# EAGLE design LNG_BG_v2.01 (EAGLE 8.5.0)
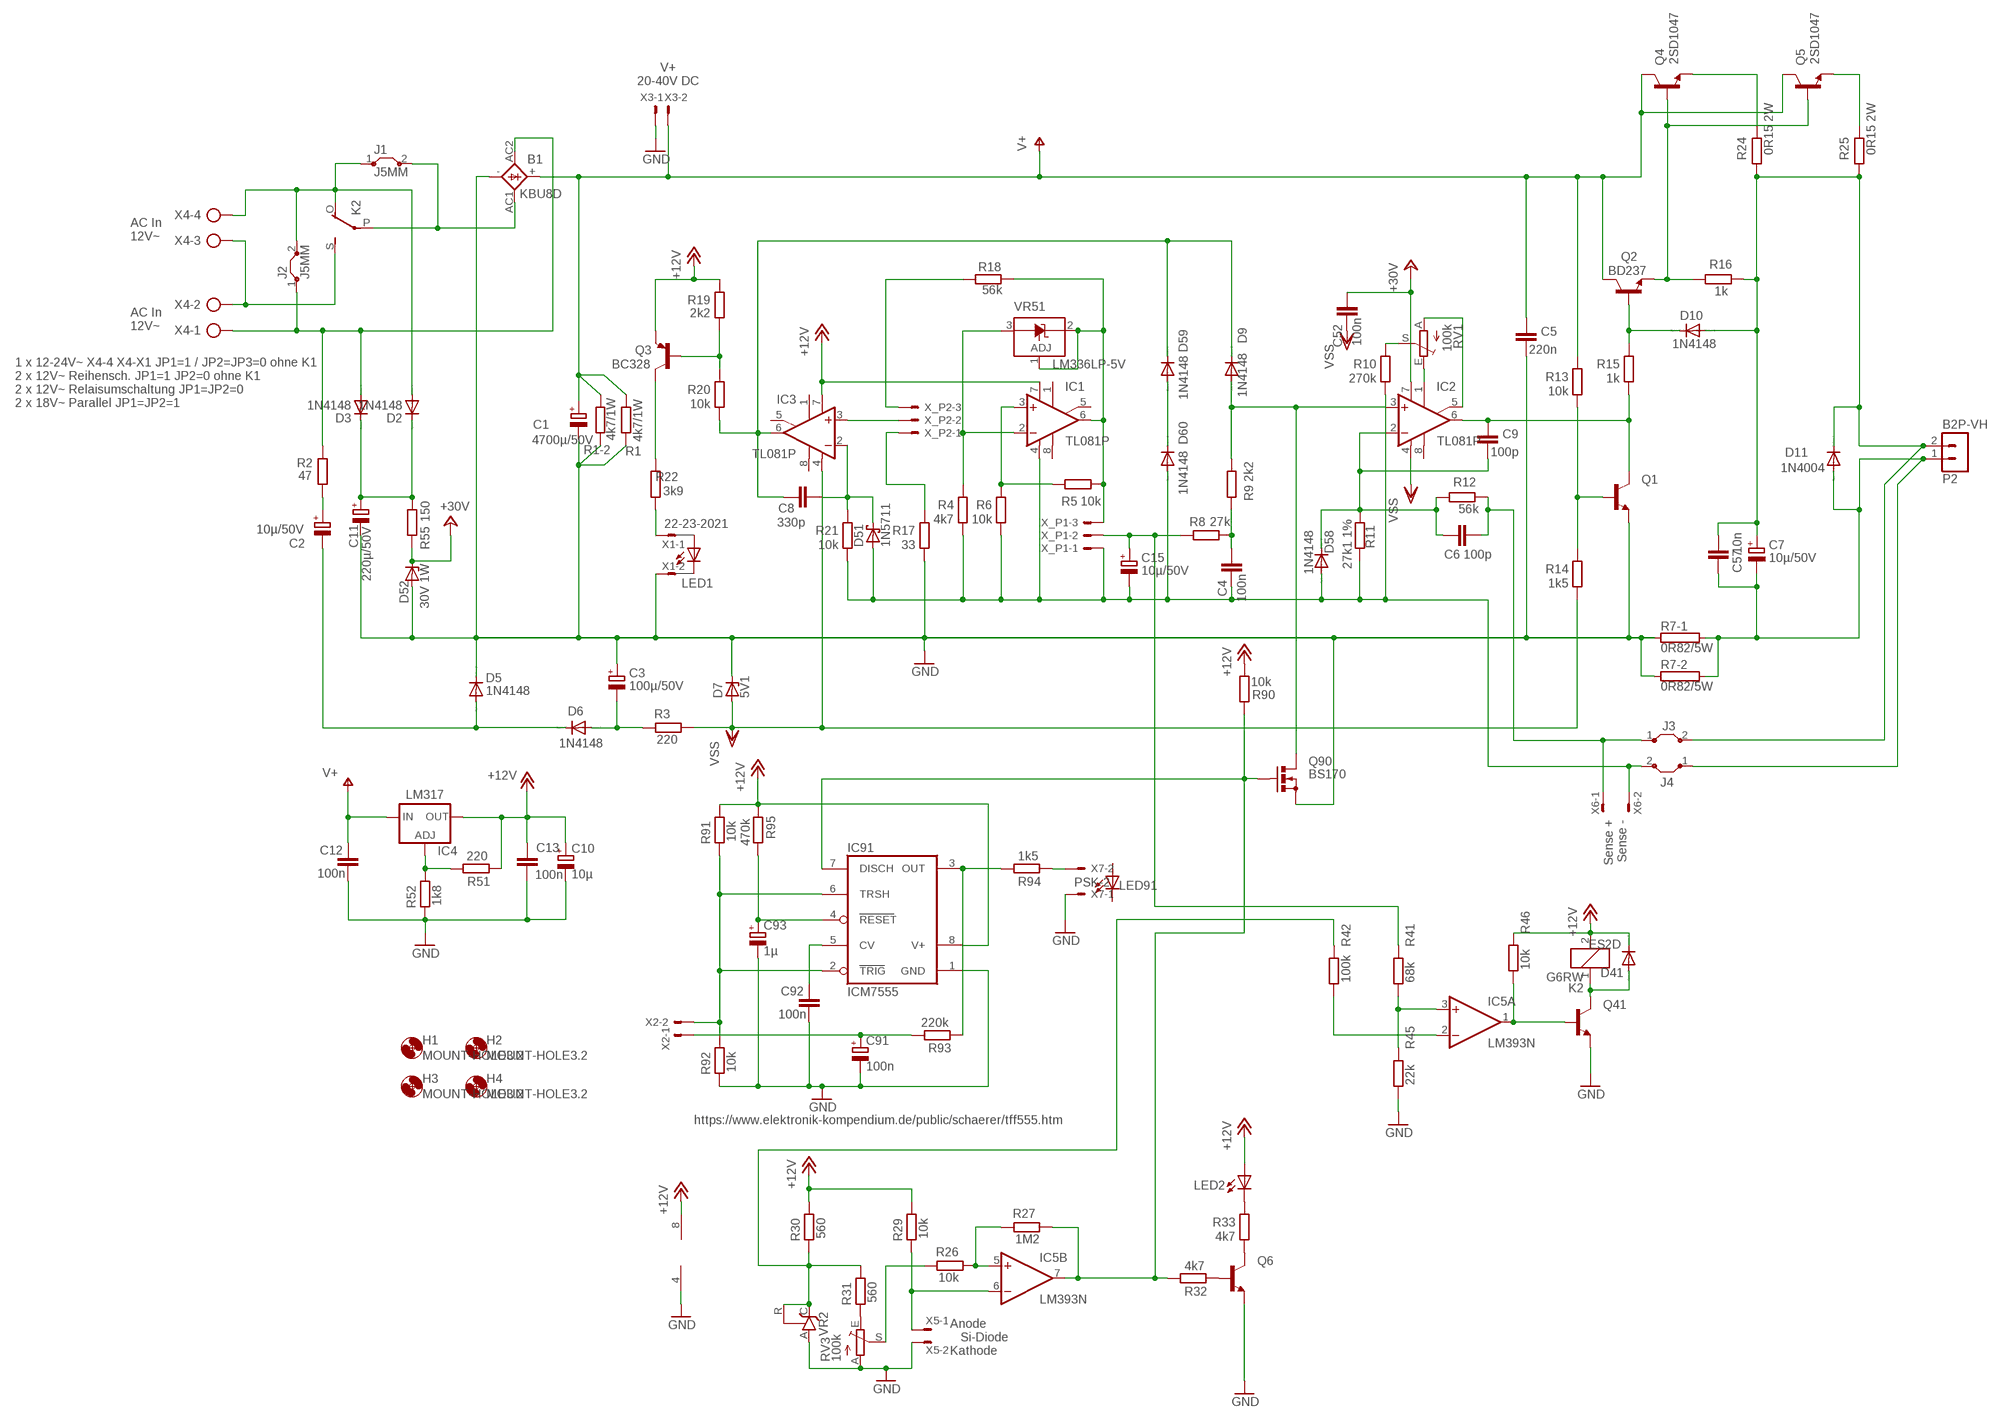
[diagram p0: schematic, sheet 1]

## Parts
B1  KBU8D  GBU4  [GBU4S]
C1  4700µ/50V  CPOL-EUE10-25  [EB25D]
C2  10µ/50V  CPOL-EUE2.5-6  [E2,5-6]
C3  100µ/50V  CPOL-EUE2.5-6  [E2,5-6]
C4  100n  C-EU050-024X044  [C050-024X044]
C5  220n  C-EUC1206  [C1206]
C6  100p  C-EU050-024X044  [C050-024X044]
C7  10µ/50V  CPOL-EUE2.5-6  [E2,5-6]
C8  330p  C-EU050-024X044  [C050-024X044]
C9  100p  C-EU050-024X044  [C050-024X044]
C10  10µ  CPOL-EUE1.8-4  [E1,8-4]
C11  220µ/50V  CPOL-EUE5-10.5  [E5-10,5]
C12  100n  C-EUC0805K  [C0805K]
C13  100n  C-EUC0805K  [C0805K]
C15  10µ/50V  CPOL-EUE2.5-6  [E2,5-6]
C52  100n  C-EUC1206K  [C1206K]
C57  10n  C-EU050-024X044  [C050-024X044]
C91  100n  CPOL-EUE1.8-4  [E1,8-4]
C92  100n  C-EU050-024X044  [C050-024X044]
C93  1µ  CPOL-EUE1.8-4  [E1,8-4]
D2  1N4148  1N4004  [DO41-10]
D3  1N4148  1N4004  [DO41-10]
D5  1N4148  1N4148DO35-10  [DO35-10]
D6  1N4148  1N4148DO35-10  [DO35-10]
D7  5V1  BZV10  [DO34Z7]
D9  1N4148  1N4148DO35-10  [DO35-10]
D10  1N4148  1N4148DO35-10  [DO35-10]
D11  1N4004  [DO41-10]
D41  ES2D  [SMB]
D51  1N5711  SCHOTTKY-DIODEDO35-7  [DO35-7]
D52  30V 1W  ZPY  [DO41Z10]
D58  1N4148  1N4148DO35-10  [DO35-10]
D59  1N4148  1N4148DO35-10  [DO35-10]
D60  1N4148  1N4148DO35-10  [DO35-10]
H1  MOUNT-HOLE3.2  [3,2]
H2  MOUNT-HOLE3.2  [3,2]
H3  MOUNT-HOLE3.2  [3,2]
H4  MOUNT-HOLE3.2  [3,2]
IC1  TL081P  [DIL08]
IC2  TL081P  [DIL08]
IC3  TL081P  [DIL08]
IC4  LM317  LM317TS  [317TS]
IC5  LM393N  [DIL08]
IC91  ICM7555  [DIL08]
J1  J5MM  [05]
J2  J5MM  [05]
J3  J5MM  [05]
J4  J5MM  [05]
K2  G6RW  [G6RW]
LED1  LED3MM  [LED3MM]
LED2  LED3MM  [LED3MM]
LED91  LED3MM  [LED3MM]
P2  B2P-VH  [B2P-VH]
Q1  BC337-NPN-TO92-CBE  [TO92-CBE]
Q2  BD237  -NPN-TO126V  [TO126V]
Q3  BC328  [TO92-EBC]
Q4  2SD1047  2SC3855  [SC-65]
Q5  2SD1047  2SC3855  [SC-65]
Q6  BC337-NPN-TO92-CBE  [TO92-CBE]
Q41  BC337-NPN-TO92-CBE  [TO92-CBE]
Q90  BS170  [SOT54E]
R1  4k7/1W  R-EU_R2512  [R2512]
R1-2  4k7/1W  R-EU_R2512  [R2512]
R2  47  R-EU_0207/10  [0207/10]
R3  220  R-EU_0207/10  [0207/10]
R4  4k7  R-EU_0207/10  [0207/10]
R5  10k  R-EU_0207/10  [0207/10]
R6  10k  R-EU_0207/10  [0207/10]
R7-1  0R82/5W  RKH208-8  [KH208-8]
R7-2  0R82/5W  RKH208-8  [KH208-8]
R8  27k  R-EU_0207/10  [0207/10]
R9  2k2  R-EU_0207/10  [0207/10]
R10  270k  R-EU_0207/10  [0207/10]
R11  27k1 1%  R-EU_0207/10  [0207/10]
R12  56k  R-EU_0207/10  [0207/10]
R13  10k  R-EU_0207/10  [0207/10]
R14  1k5  R-EU_0207/10  [0207/10]
R15  1k  R-EU_0207/10  [0207/10]
R16  1k  R-EU_0207/10  [0207/10]
R17  33  R-EU_0207/10  [0207/10]
R18  56k  R-EU_0207/10  [0207/10]
R19  2k2  R-EU_0207/10  [0207/10]
R20  10k  R-EU_0207/10  [0207/10]
R21  10k  R-EU_0207/10  [0207/10]
R22  3k9  R-EU_0207/10  [0207/10]
R24  0R15 2W  R-EU_0613/15  [P0613/15]
R25  0R15 2W  R-EU_0613/15  [P0613/15]
R26  10k  R-EU_0207/10  [0207/10]
R27  1M2  R-EU_0207/10  [0207/10]
R29  10k  R-EU_0207/10  [0207/10]
R30  560  R-EU_0207/10  [0207/10]
R31  560  R-EU_0207/10  [0207/10]
R32  4k7  R-EU_0207/10  [0207/10]
R33  4k7  R-EU_0207/10  [0207/10]
R41  68k  R-EU_0207/10  [0207/10]
R42  100k  R-EU_0207/10  [0207/10]
R45  22k  R-EU_0207/10  [0207/10]
R46  10k  R-EU_0207/10  [0207/10]
R51  220  R-EU_0207/10  [0207/10]
R52  1k8  R-EU_0207/10  [0207/10]
R55  150  R-EU_0207/10  [0207/10]
R90  10k  R-EU_0207/10  [0207/10]
R91  10k  R-EU_0207/10  [0207/10]
R92  10k  R-EU_0207/10  [0207/10]
R93  220k  R-EU_0207/10  [0207/10]
R94  1k5  R-EU_0207/10  [0207/10]
R95  470k  R-EU_0207/10  [0207/10]
RV1  100k  TRIM_EU-B64Y  [B64Y]
RV3  100k  TRIM_EU-B64Y  [B64Y]
VR2  TL431CLP  [TO92-CLP]
VR51  LM336LP-5V  LM336LP  [TO92]
X1  22-23-2021  [22-23-2021]
X2  PSK-2  22-23-2021  [22-23-2021]
X3  PSK-2  22-23-2021  [22-23-2021]
X4  AK500/4  [AK500/4]
X5  PSK-2  22-23-2021  [22-23-2021]
X6  22-23-2021  [22-23-2021]
X7  PSK-2  22-23-2021  [22-23-2021]
X_P1  22-23-2031  [22-23-2031]
X_P2  22-23-2031  [22-23-2031]

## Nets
+12V: C10.+ C13.1 D41.C IC1.7(V+) IC3.7(V+) IC4.2(OUT) IC5.8(P:V+) IC91.8(V+) K2.2 LED2.A Q3.E R19.2 R29.2 R30.2 R46.2 R51.1 R90.1 R91.2 R95.1
+24V: C52.1 D52.C IC2.7(V+) R55.1 ; supply symbol labelled +30V
+SENSE: C7.+ C57.2 D10.A D11.C J3.2 P2.2 R16.1 R24.2 R25.2
-SENSE: C4.2 C15.- D51.A D58.A D60.A IC1.4(V-) J4.2 R4.1 R6.1 R10.1 R11.1 R21.1 X6.2 X_P1.1
AC2-1: K2.S(2:S) X4.2 X4.3
AC2-2: B1.AC2(AC1) D3.A J2.1 R2.1 X4.1
GND: B1.- C1.- C3.+ C5.2 C10.- C11.- C12.2 C13.2 C91.- C92.2 C93.- D5.C D7.C D52.A IC5.4(P:V-) IC91.1(GND) Q1.E Q6.E Q41.E Q90.S R1-2.1 R1.1 R7-1.1 R7-2.1 R17.1 R45.1 R52.1 R92.1 RV3.A VR2.A X1.2 X3.1 X5.2 X7.1
N$1: IC91.3(OUT) R93.1 R94.2
N$2: R94.1 X7.2
N$3: C2.+ R2.2
N$4: B1.AC1(AC2) J1.2 K2.P(2:P)
N$5: C2.- D5.A D6.C
N$6: Q3.B R19.1 R20.2
N$7: C3.- D6.A R3.1
N$8: D59.A D60.C
N$9: C8.2 D9.C D59.C IC3.6(OUT) R20.1
N$10: C8.1 D51.C IC3.2(-IN) R21.2
N$11: R22.1 X1.1
N$12: Q3.C R22.2
N$13: C11.+ D2.C D3.C R55.2
N$14: IC3.3(+IN) X_P2.2
N$15: R17.2 X_P2.1
N$16: R18.2 X_P2.3
N$17: IC1.3(+IN) R5.2 R6.2
N$18: C15.+ R8.2 R41.2 X_P1.2
N$19: IC1.2(-IN) R4.2 VR51.3(A)
N$21: C4.1 R8.1 R9.2
N$22: D9.A IC2.3(+IN) Q90.D R9.1
N$23: C93.+ IC91.4(RESET) R95.2
N$24: R10.2 RV1.S
N$25: IC2.1(ON1) RV1.E
N$26: IC2.5(ON2) RV1.A
N$27: C9.1 IC2.6(OUT) Q1.C R15.1
N$28: Q1.B R13.1 R14.2
N$29: D10.C Q2.3(B) R15.2
N$30: IC5.3(A:+IN) R41.1 R45.2
N$31: IC5.5(B:+IN) R26.2 R27.1
N$32: IC91.2(TRIG) IC91.6(TRSH) R91.1 R92.2 X2.2
N$33: IC5.2(A:-IN) R42.1
N$35: C6.1 C9.2 D58.C IC2.2(-IN) R11.2 R12.2
N$36: C92.1 IC91.5(CV)
N$37: IC5.6(B:-IN) R29.1 X5.1
N$39: IC5.1(A:OUT) Q41.B R46.1
N$40: R30.1 R31.2 R42.2 VR2.C VR2.R
N$41: D41.A K2.1 Q41.C
N$42: Q4.3(E) R24.1
N$43: R31.1 RV3.E
N$44: IC4.1(ADJ) R51.2 R52.2
N$45: R26.1 RV3.S
N$46: D2.A J1.1 J2.2 K2.O(2:O) X4.4
N$48: C6.2 J3.1 R12.1 X6.1
N$50: Q2.1(E) Q4.1(B) Q5.1(B) R16.2
N$51: Q5.3(E) R25.1
N$53: C91.+ R93.2 X2.1
N$54: Q6.B R32.1
N$55: C7.- C57.1 D11.A J4.1 P2.1 R7-1.2 R7-2.2
N$56: Q6.C R33.1
N$57: LED2.K(C) R33.2
N$58: IC5.7(B:OUT) IC91.7(DISCH) Q90.G R27.2 R32.2 R90.2
V+: B1.+ C1.+ C5.1 C12.1 IC4.3(IN) Q2.2(C) Q4.2(C) Q5.2(C) R1-2.2 R1.2 R13.2 X3.2
VREF: IC1.6(OUT) R5.1 R18.1 VR51.1(ADJ) VR51.2(C) X_P1.3
VSS: C52.2 D7.A IC2.4(V-) IC3.4(V-) R3.2 R14.1
Unconnected: IC1.1(ON1) IC1.5(ON2) IC1.8(OPT) IC2.8(OPT) IC3.1(ON1) IC3.5(ON2) IC3.8(OPT) LED1.A LED1.K(C) LED91.A LED91.K(C)

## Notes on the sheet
- V+
  20-40V DC
- AC In
  12V~
- AC In
  12V~
- 1 x 12-24V~ X4-4 X4-X1 JP1=1 / JP2=JP3=0 ohne K1
  2 x 12V~ Reihensch. JP1=1 JP2=0 ohne K1
  2 x 12V~ Relaisumschaltung JP1=JP2=0
  2 x 18V~ Parallel JP1=JP2=1
- Sense +
  Sense -
- https://www.elektronik-kompendium.de/public/schaerer/tff555.htm
- Anode
     Si-Diode
  Kathode

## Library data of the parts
B1 = rectifier:GBU4: GENERAL INSTRUMENT RECTIFIER
C1-C3 C7 C10 C11 C15 C91 C93 = rcl:CPOL-EU: POLARIZED CAPACITOR, European symbol; SPICEPREFIX: C
C4-C6 C8 C9 C12 C13 C52 C57 C92 = rcl:C-EU: CAPACITOR, European symbol; SPICEPREFIX: C
D2 D3 D11 = diode:1N4004: DIODE
D5 D6 D9 D10 D58-D60 = diode:1N4148: DIODE
D7 = diode:BZV10: Z DIODE
D41 = diode:ES2D: DIODE
D51 = diode:SCHOTTKY-DIODE: Schottky Diode
D52 = diode:ZPY: Z DIODE
H1-H4 = holes:MOUNT-HOLE: MOUNTING HOLE with drill center marker
IC1-IC3 = linear:TL081: OP AMP
IC4 = v-reg:LM317TS: VOLTAGE REGULATOR
IC5 = linear:LM393: COMPARATOR
IC91 = maxim:ICM7555: TIMER; MF: MAXIM; MPN: ICM7555IPA+; OC_FARNELL: 9663762; OC_NEWARK: 68K4387
J1-J4 = jumper:J: Bridge
K2 = relay:G6RW: RELAY 1 x switch, Omron; OC_FARNELL: unknown; OC_NEWARK: unknown
LED1 LED2 LED91 = led:LED: LED
P2 = con-jst-vh:B2P-VH: HEADER
Q1 Q2 Q6 Q41 = transistor:*-NPN-: NPN Transistror BF959 corrected 2008.03.06
Q3 = transistor-pnp:BC328*: PNP Transistror
Q4 Q5 = transistor-JP:2SC3855: NPN Power Transistor 140V, 10A, 100W
Q90 = transistor-small-signal:BS170: N-CHANNEL MOS FET
R1 R1-2 R2-R6 R8-R22 R24-R27 R29-R33 R41 R42 R45 R46 R51 R52 R55 R90-R95 = rcl:R-EU_: RESISTOR, European symbol; SPICEPREFIX: R
R7-1 R7-2 = resistor-power:R: Power Resitor; OC_FARNELL: unknown; OC_NEWARK: unknown
RV1 RV3 = pot:TRIM_EU-: POTENTIOMETER
VR2 = v-reg:TL431CLP: VOLTAGE REGULATOR
VR51 = linear:LM336: 2.5-V INTEGRATED REFERENCE CIRCUITS LM236 Source: http://focus.ti.com/lit/ds/symlink/lm336-2.5.pdf
X1-X3 X5-X7 = con-molex:22-23-2021: .100" (2.54mm) Center Header - 2 Pin; MF: MOLEX; MPN: 22-23-2021; OC_FARNELL: 1462926; OC_NEWARK: 25C3832
X4 = con-ptr500:AK500/4: CONNECTOR; OC_FARNELL: unknown; OC_NEWARK: unknown
X_P1 X_P2 = con-molex:22-23-2031: .100" (2.54mm) Center Header - 3 Pin; MF: MOLEX; MPN: 22-23-2031; OC_FARNELL: 1462950; OC_NEWARK: 30C0862

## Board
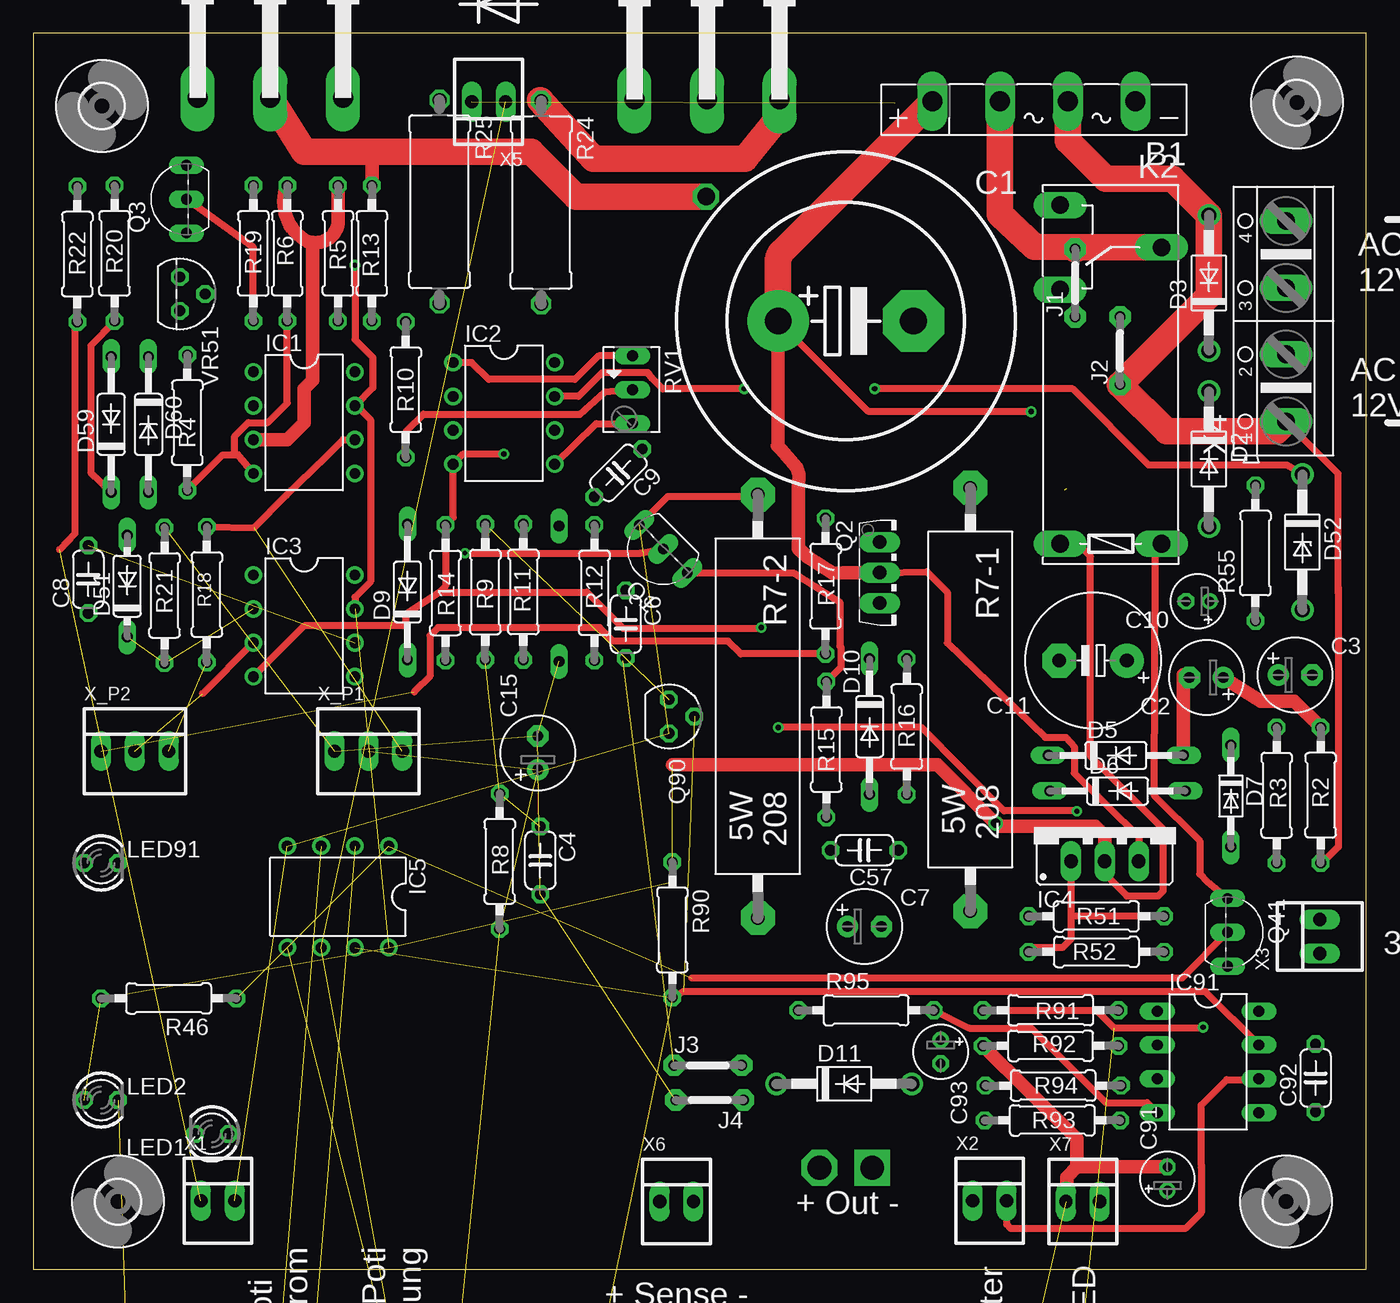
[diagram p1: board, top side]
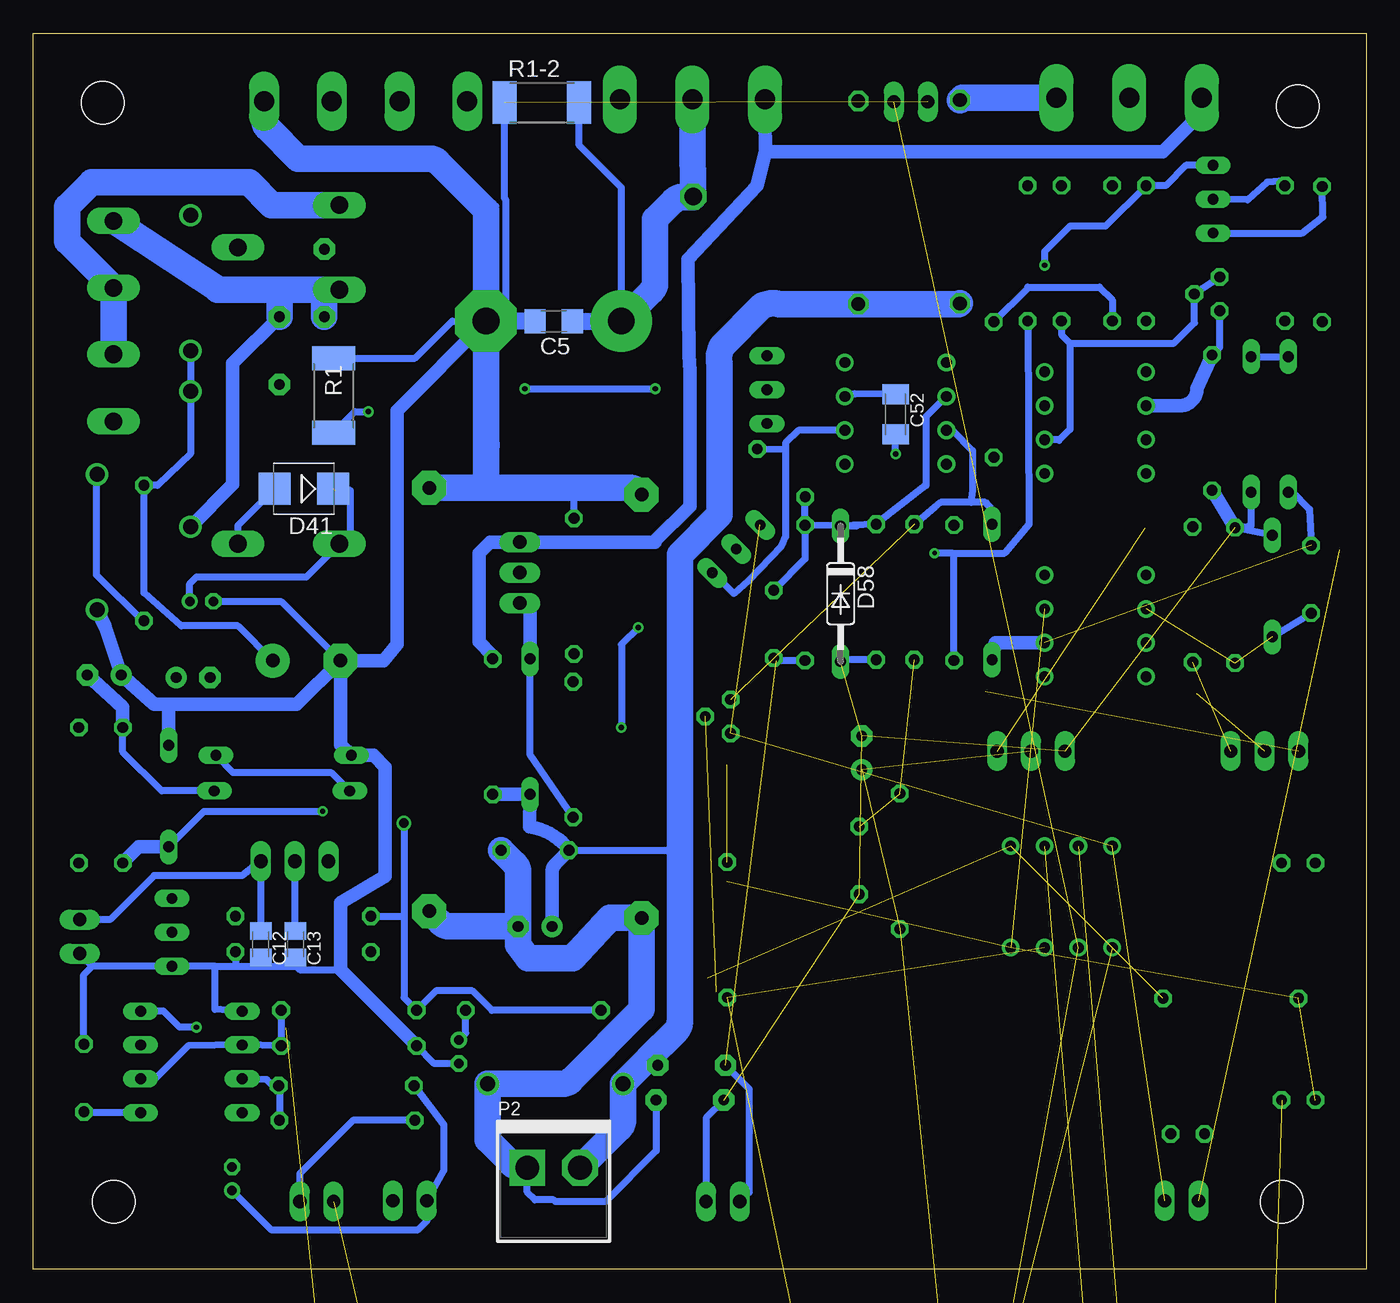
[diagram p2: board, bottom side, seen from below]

Size 100 x 92.7 mm. Coordinates in mm from the lower left corner, seen from the top.
Outline: 0,0 100,0 100,92.7 0,92.7 0,0
Copper layers (1*16): Top 0.035mm / dielectric 1.5mm / Bottom 0.035mm
Design rules "default *": minimum track width 6mil, minimum drill 0.35mm, track to track 10mil, track to pad 10mil, pad to pad 10mil, via to via 15mil, smd to smd 6mil, copper to edge 40mil, drill to drill 6mil, minimum pad ring 10mil, minimum via ring 8mil, stop-mask expansion 4mil, vias tented up to drill 0mil, thermal gap 10mil

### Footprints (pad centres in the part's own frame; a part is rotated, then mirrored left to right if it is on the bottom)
GBU4S = drill 1.499 long: + 7.62,0; - -7.62,0; AC1 2.54,0; AC2 -2.54,0
EB25D = drill 2.007 pad 4.597: + -5.08,0 | drill 2.007 pad 4.597 octagon: - 5.08,0
E2,5-6 = drill 0.813 pad 1.6: + -1.27,0 | drill 0.813 pad 1.6 octagon: - 1.27,0
C050-024X044 = drill 0.813 octagon: 1 -2.54,0; 2 2.54,0
C1206 = smd 1.6 x 1.8: 1 -1.4,0; 2 1.4,0
E1,8-4 = drill 0.711 pad 1.168: + -0.889,0 | drill 0.711 pad 1.168 octagon: - 0.889,0
E5-10,5 = drill 1.016 pad 2.54: + -2.54,0 | drill 1.016 pad 2.54 octagon: - 2.54,0
C0805K = smd 1.3 x 1.6: 1 -1,0; 2 1,0
C1206K = smd 1.5 x 2: 1 -1.5,0; 2 1.5,0
DO41-10 = drill 1.118: A 5.08,0; C -5.08,0
DO35-10 = drill 0.813 long: A 5.08,0; C -5.08,0
DO34Z7 = drill 0.813 long: A 3.81,0; C -3.81,0
SMB = smd 2.4 x 2.4: A 2.2,0; C -2.2,0
DO35-7 = drill 0.813 long: A 3.81,0; C -3.81,0
DO41Z10 = drill 1.118: A 5.08,0; C -5.08,0
3,2 = hole 3.2: 0,0
DIL08 = drill 0.813 pad 1.27: 1 -3.81,-3.81; 2 -1.27,-3.81; 3 1.27,-3.81; 4 3.81,-3.81; 5 3.81,3.81; 6 1.27,3.81; 7 -1.27,3.81; 8 -3.81,3.81
317TS = drill 1.016 long: 1 -2.54,-2.54; 2 0,-2.54; 3 2.54,-2.54
DIL08' = drill 0.813 long: 1 -3.81,-3.81; 2 -1.27,-3.81; 3 1.27,-3.81; 4 3.81,-3.81; 5 3.81,3.81; 6 1.27,3.81; 7 -1.27,3.81; 8 -3.81,3.81
05 = drill 0.813 pad 1.6 octagon: 1 -2.54,0; 2 2.54,0
G6RW = drill 1.321 long: 1 -12.7,-3.81; 2 -12.7,3.81; O 6.35,3.81; P 9.525,-3.81; S 12.7,3.81
LED3MM = drill 0.813 octagon: A -1.27,0; K 1.27,0
B2P-VH = drill 1.778 square: 1 -1.98,0 | drill 1.778 octagon: 2 1.98,0
TO92-CBE = drill 0.813 long: B 0,0; C -2.54,0; E 2.54,0
TO126V = drill 1.016 long: 1 -2.286,-1.27; 2 0,-1.27; 3 2.286,-1.27
TO92-EBC = drill 0.813 long: B 0,-1.27; C -2.54,-1.27; E 2.54,-1.27
SC-65 = drill 1.5 pad 2.54 long: 1 -5.45,-18.81; 2 0,-18.81; 3 5.45,-18.81
SOT54E = drill 0.813 octagon: D -1.27,0; G 0,1.905; S 1.27,0
R2512 = smd 1.8 x 3.2: 1 -2.8,0; 2 2.8,0
0207/10 = drill 0.813 octagon: 1 -5.08,0; 2 5.08,0
KH208-8 = drill 1.016 pad 2.54 octagon: 1 -15.875,0; 2 15.875,0
P0613/15 = drill 1.016 octagon: 1 -7.62,0; 2 7.62,0
B64Y = drill 0.813 long: A 2.54,0; E -2.54,0; S 0,0
TO92-CLP = drill 0.813 octagon: A 0,1.905; C 1.27,0; R -1.27,0
TO92 = drill 0.813 octagon: 1 -1.27,0; 2 0,1.905; 3 1.27,0
22-23-2021 = drill 1 long: 1 -1.27,0; 2 1.27,0
AK500/4 = drill 1.321 long: 1 -7.518,0; 2 -2.489,0; 3 2.489,0; 4 7.518,0
22-23-2031 = drill 1 long: 1 -2.54,0; 2 0,0; 3 2.54,0

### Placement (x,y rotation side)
B1  75.07,87.61 180 top
C1  60.96,71.12 0 top
C2  88.01,44.39 180 top
C3  94.68,44.58 0 top
C4  38.04,30.67 270 top
C5  60.96,71.12 180 bottom
C6  44.45,48.39 270 top
C7  62.36,25.72 0 top
C8  4.13,51.75 90 top
C9  43.89,59.73 225 top
C10  87.38,50.1 180 top
C11  79.5,45.66 180 top
C12  82.93,24.38 270 bottom
C13  80.33,24.38 270 bottom
C15  37.85,38.73 90 top
C52  35.31,64.14 270 bottom
C57  62.36,31.43 180 top
C91  85.09,6.79 90 top
C92  96.2,14.35 90 top
C93  68.07,16.32 270 top
D2  88.2,60.77 270 top
D3  88.2,73.98 90 top
D5  81.22,38.54 0 top
D6  81.34,35.88 0 top
D7  89.85,35.5 270 top
D9  28.07,50.8 90 top
D10  62.74,40.7 270 top
D11  60.83,13.91 0 top
D41  79.69,58.55 180 bottom
D51  7.05,51.24 90 top
D52  95.21,54.54 270 top
D58  39.43,50.67 270 bottom
D59  5.84,63.37 90 top
D60  8.64,63.37 270 top
H1  5.14,87.25 0 top
H2  6.35,5.08 0 top
H3  93.98,5.08 0 top
H4  94.81,87.5 0 top
IC1  20.32,63.5 270 top
IC2  35.31,64.2 270 top
IC3  20.32,48.26 270 top
IC4  80.39,33.15 0 top
IC5  22.86,27.94 180 top
IC91  ICM7555  [DIL08']  88.14,15.56 270 top
J1  78.17,73.98 90 top
J2  81.53,68.9 90 top
J3  50.61,15.3 0 top
J4  50.74,12.7 180 top
K2  80.84,67.12 90 top
LED1  13.4,10.16 180 top
LED2  5.08,12.7 0 top
LED91  5.08,30.48 0 top
P2  60.96,7.62 0 bottom
Q1  47.26,54.03 135 top
Q2  64.77,52.26 270 top
Q3  10.22,80.26 90 top
Q4  50.55,106.55 0 top
Q5  17.78,106.68 0 top
Q6  not placed on the board
Q41  89.6,25.27 270 top
Q90  47.69,41.47 270 top
R1  77.47,65.53 270 bottom
R1-2  61.85,87.5 0 bottom
R2  96.58,35.56 90 top
R3  93.28,35.56 270 top
R4  11.56,63.5 90 top
R5  22.86,76.2 90 top
R6  19.05,76.2 90 top
R7-1  70.29,42.74 270 top
R7-2  54.36,42.23 270 top
R8  34.99,30.61 270 top
R9  33.91,50.8 270 top
R10  27.94,65.98 270 top
R11  36.77,50.8 90 top
R12  42.1,50.74 90 top
R13  25.4,76.2 90 top
R14  30.92,50.74 270 top
R15  59.5,38.99 270 top
R16  65.53,40.7 90 top
R17  59.44,51.24 270 top
R18  13.02,50.61 270 top
R19  16.51,76.2 90 top
R20  6.1,76.2 90 top
R21  9.84,50.55 270 top
R22  3.3,76.14 90 top
R24  38.1,80.01 270 top
R25  30.48,80.07 270 top
R26  not placed on the board
R27  not placed on the board
R29  not placed on the board
R30  not placed on the board
R31  not placed on the board
R32  not placed on the board
R33  not placed on the board
R41  not placed on the board
R42  not placed on the board
R45  not placed on the board
R46  10.16,20.32 180 top
R51  79.76,26.48 0 top
R52  79.76,23.81 180 top
R55  91.69,53.72 90 top
R90  47.94,25.46 270 top
R91  76.33,19.43 180 top
R92  76.33,16.76 0 top
R93  76.52,13.78 180 top
R94  76.45,11.18 0 top
R95  62.48,19.43 0 top
RV1  44.96,65.98 270 top
RV3  not placed on the board
VR2  not placed on the board
VR51  10.99,73.15 270 top
X1  13.84,5.14 0 top
X2  71.75,5.14 0 top
X3  96.52,24.96 90 top
X4  93.98,71.12 90 top
X5  34.16,87.57 180 top
X6  48.26,5.08 0 top
X7  78.74,5.08 0 top
X_P1  25.15,38.86 0 top
X_P2  7.62,38.86 0 top

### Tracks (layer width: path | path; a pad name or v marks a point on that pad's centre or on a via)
+12V  (via drill 0.4, 0.7)  (8 unrouted)
  Top 0.508: IC3.7 24.13,50.42 25.3,51.59 25.3,63.73 24.13,64.9 IC1.7 25.46,66.1 25.46,68.39 24.13,69.72 v24.13,75.31 | 47.94,29.08 R90.1 | R91.2 79.75,19.43 81.05,18.14 87.73,18.14 v87.76,18.16 | IC4.2 80.39,29.66 82.04,28 84.39,28 84.77,28.38 84.77,33.02 79.31,38.48 79.31,53.47 78.3,54.48 78.23,54.42 K2.2
  Top 1.016: IC4.2 80.39,32.51 79.69,33.21 72.57,33.21 72.32,33.46 v72.2,33.46 67.82,37.85 47.94,37.85
  Bottom 0.508: Q3.E 13.53,82.8 15.05,81.28 R19.2 19.56,78.23 22.23,78.23 24.13,76.33 v24.13,75.31 | 77.36,58.42 76.2,58.42 76.2,55.24 K2.2 79.5,51.94 87.76,51.94 88.27,51.43 C10.+ | 70.93,19.43 R91.2 | IC4.2 80.39,25.45 C13.1 | R91.2 72.2,20.38 72.2,26.42 | v72.2,33.46 72.2,26.42 | R95.1 65.6,19.43 67.06,20.89 69.79,20.89 R91.2 | v87.76,18.16 89.03,18.16 90.23,19.37 IC91.8 | R51.1 72.26,26.48 72.2,26.42
+24V  (via drill 0.4)
  Top 0.508: v53.34,66.04 47.21,66.04 46.46,66.78 46.1,67.25 42.67,67.25 40.89,65.47 IC2.7 | v63.12,66.04 77.98,66.04 83.69,60.32 94.07,60.32 D52.C
  Bottom 0.508: v63.12,66.04 v53.34,66.04 | C52.1 38.35,65.66 IC2.7 | R55.1 91.69,48.51 95.25,52.07 95.25,58.33 D52.C
+SENSE
  Bottom 0.508: C57.2 52.45,31.43 51.5,30.48 | 51.37,45.85 51.5,45.72 | J3.2 53.4,15.3 53.88,15.78
  Bottom 1.016: R16.1 D10.A 62.78,33.19 arc45 59.75,31.4 C57.2 60.79,30.45 arc-45 61.09,29.75 C7.+
  Bottom 2: P2.2 56.05,10.55 arc-45 55.75,11.26 D11.C 53.88,15.78 51.79,17.87 arc-45 51.5,18.57 51.5,30.48 51.5,45.72 51.5,53.59 48.51,56.58 48.51,67.97 arc45 48.32,69.22 45.38,72.22 arc45 44.04,72.39 R24.2 30.63,72.39 arc-45 R25.2
-SENSE  (5 unrouted)
  Top 0.508: IC1.4 15.24,61.15 15.18,61.15 15.11,61.09 | 15.11,61.09 15.11,62.48 16.13,63.5 17.59,63.5 19.05,64.96 R6.1 | R4.1 14.22,61.09 15.11,61.09
  Bottom 0.508: D60.A 8.64,55.75 R21.1 D51.A | R10.1 25.4,73.6 25.4,73.66 20,73.66 19.05,72.71 R6.1 | R11.1 39.31,45.72 D58.A | J4.2 49.53,11.37 X6.2
  Bottom 1.016: R21.1 R4.1
AC2-1
  Bottom 2: X4.2 X4.3 97.47,77.1 97.47,79.69 95.63,81.53 83.82,81.53 82.11,79.82 K2.S
AC2-2
  Top 0.508: 97.88,51.69 97.89,50.78 | 97.89,50.78 97.92,49.68 97.92,31.69 96.71,30.48 R2.1 | 97.89,50.78 97.89,59.69 X4.1
  Top 2: B1.AC2 77.61,84.64 80.45,81.79 85.47,81.79 D3.A 88.2,73.02 J2.1 85.05,62.84 89.85,62.86 93.24,62.86 X4.1
GND  (8 unrouted)
  Top 0.508: Q1.E 47.62,57.98 53.78,57.98 R7-2.1 | X7.1 77.53,5.14
  Top 1.016: 77.53,5.14 77.53,6.92 78.3,7.68 | 78.3,7.68 C91.- | R92.1 78.3,9.78 78.3,7.68
  Bottom 0.508: 65.31,79.73 arc45 66.02,79.44 66.04,79.44 | 65.98,61.85 arc-90 66.04,61.79 | 89.53,22.8 Q41.E | R17.1 59.44,58.42 59.24,58.61 | Q41.E 95.57,22.73 | 95.57,22.73 X3.1 | R1-2.1 64.65,80.33 64.58,80.26 64.58,72.58 C1.- 68.58,71.12 71.37,68.33 R1.1 | 86.36,22.73 Q41.E | IC91.1 86.36,19.49 86.36,22.73 | 70.8,16.76 R92.1 69.91,15.43 C93.- | C92.2 96.2,22.1 95.57,22.73 | 80.39,22.86 80.39,22.73 83,22.73 | 80.39,22.86 80.39,23.32 C13.2 | 86.36,22.73 84.9,22.73 | 84.9,22.73 83,22.73 | C12.2 83,23.32 83,22.73 | 80.39,22.86 80.01,22.48 76.96,22.48 | R52.1 84.84,22.8 84.9,22.73 | C10.- 81.41,50.1 C11.-
  Bottom 1.016: 54.36,58.45 R7-2.1 | C1.- 72.71,64.39 72.71,46.86 73.72,45.66 76.95,45.66 | C11.- 76.95,45.66 | 76.95,45.66 80.23,42.37 89.92,42.37 | 89.92,42.37 90.95,42.37 C3.+ 94.61,48.2 94.62,48.2 D52.A | D7.C 89.85,42.3 89.92,42.37 | 76.95,45.66 76.95,39.35 D5.C 74.49,38.55 73.6,37.66 73.6,29.46 76.96,27.5 76.96,22.48 R92.1
  Bottom 1.27: C5.2 C1.-
  Bottom 2: B1.- 82.69,86.27 arc-45 82.39,85.57 80.14,83.31 70.33,83.31 arc45 69.62,83.02 66.04,79.44 C1.- 66.04,61.79 | R7-2.1 54.57,58.32 arc-45 55.28,58.61 59.24,58.61 66.04,58.61 | 66.04,58.61 R7-1.1 | 65.98,61.85 arc-45 66.04,61.7 66.04,58.61
N$1
  Bottom 0.508: R94.2 81.53,13.72 R93.1 82.04,13.78 82.49,14.22 IC91.3
N$2
  Bottom 0.508: R94.1 76.01,11.18 80.01,7.18 X7.2
N$3
  Top 1.016: C2.+ 92.08,42.61 94.61,42.61 R2.2
N$4
  Top 2: K2.P 78.23,76.64 | 78.23,76.64 75.12,76.71 72.52,79.12 72.52,87.63 72.53,87.19 B1.AC1 | J1.2 78.23,76.58 78.23,76.64
N$5
  Top 1.016: C2.- 86.3,44.58 D5.A
  Bottom 0.508: D5.A 85.03,37.27 77.66,37.27 D6.C
N$6
  Top 0.508: R19.1 16.51,76.64 Q3.B
  Bottom 0.508: R20.2 6.1,81.66 7.43,81.53 8.89,80.2 Q3.B
N$7
  Bottom 0.508: D6.A 90.36,35.88 93.28,38.8 R3.1
  Bottom 1.016: C3.- 93.28,42.16 R3.1
N$8
  Bottom 0.508: D60.C D59.A
N$9  (1 unrouted)
  Top 0.508: R20.1 4.32,69.28 4.32,59.75 D59.C
  Bottom 0.508: C8.2 4.25,57.02 5.52,58.29 D59.C
  Bottom 1.016: D9.C 27.81,46.99 IC3.6
N$10  (2 unrouted)
  Bottom 0.508: D51.C C8.1
N$11  (1 unrouted)
  Top 0.508: R22.1 3.11,70.68 3.11,55.18 1.97,53.98
N$12
  Bottom 0.508: Q3.C 4.83,77.72 3.24,78.93 R22.2
N$13
  Bottom 0.508: C11.+ 84.64,48.26 88.9,48.26 91.69,50.74 R55.2 90.68,58.8 88.2,61.15 D2.C D3.C
N$14  (1 unrouted)
  Top 0.508: 12.7,43.18 IC3.3
N$15  (1 unrouted)
  Top 0.508: 28.57,43.31 29.76,44.49 29.76,47.54 30.35,48.13 42.48,48.13 43.5,47.12 52.13,47.12 53.09,46.16 R17.2
N$16  (1 unrouted)
N$17
  Top 1.016: R5.2 22.86,78.42 arc-90 20.95,77.02 | 20.95,77.02 20.83,76.96 arc-90 R6.2 | 20.95,77.02 20.95,66.67 20.32,66.04 20.32,63.5 19.05,62.23 IC1.3
N$18  (3 unrouted)
N$19
  Bottom 0.508: R4.2 10.99,69.15 VR51.3
  Bottom 1.016: IC1.2 13.97,64.77 arc-90 12.7,66.04 R4.2
N$21  (2 unrouted)
N$22  (1 unrouted)
  Bottom 0.508: D9.A 28.07,56.96 28.57,57.53 29.65,57.53 | 29.65,57.53 31.94,57.53 32.38,57.15 R9.1 | IC2.3 31.05,62.93 29.53,61.41 29.53,58.42 29.65,57.53
N$23
  Top 0.508: R95.2 70.23,18.1 74.87,18.1 80.45,12.51 83.57,12.51 IC91.4
  Bottom 0.508: C93.+ 67.56,17.72 R95.2
N$24
  Top 0.508: RV1.S 42.86,65.79 41,64.1 29.31,64.1 29.27,64.14 27.94,62.8 R10.2
N$25
  Top 0.508: RV1.E 42.42,68.52 40.64,66.74 34.16,66.74 32.89,68.01 IC2.1
N$26
  Top 0.508: IC2.5 42.23,63.44 RV1.A
N$27  (1 unrouted)
  Top 0.508: R15.1 60.6,45.17 60.6,46.65 60.52,46.74 60.52,50.04 57.05,52.23 Q1.C
  Bottom 0.508: IC2.6 42.61,62.93 43.56,61.98 43.56,61.53 | 43.56,61.53 43.56,54.93 43.88,54.23 46.35,51.62 47.43,50.67 Q1.C | C9.1 43.56,61.53
N$28  (via drill 0.35)
  Top 0.508: v32.38,53.72 45.53,53.72 Q1.B
  Bottom 0.508: R13.1 25.3,55.88 27.05,53.78 27.11,53.72 31.05,53.72 | 31.05,53.72 v32.38,53.72 | R14.2 30.92,53.59 31.05,53.72
N$29
  Bottom 0.508: R15.2 62.74,38.61 D10.C
  Bottom 1.016: D10.C 62.74,49.98 Q2.3
N$30  (2 unrouted)
N$31  (2 unrouted)
N$32
  Top 0.508: X2.2 73.03,3.37 73.34,3.05 86.42,3.05 87.63,4.25 87.63,7.62 87.63,7.87 87.63,12.32 89.53,14.22 91.89,14.22 IC91.6
  Bottom 0.508: IC91.6 90.93,14.22 88.39,16.76 IC91.2 R92.2 R91.1
N$33  (1 unrouted)
N$35
  Bottom 0.508: IC2.2 33.02,63.94 33.02,58.8 R11.2 D58.C 38.23,55.75 R12.2 | R12.2 C9.2 | R12.2 42.1,53.28 C6.1
N$36
  Bottom 0.508: IC91.5 96.14,11.75 C92.1
N$37  (2 unrouted)
N$39  (2 unrouted)
  Top 0.508: Q41.B 86.17,21.84 49.4,21.84
N$40  (4 unrouted)
N$41
  Top 0.508: Q41.C 88.08,29.08 87.5,29.66 87.5,32.13 84.08,35.56 84.14,53.91 K2.1
  Bottom 0.508: K2.1 84.64,55.79 D41.A
N$42
  Top 2: Q4.3 56,86.48 53.4,83.31 42.02,83.31 38.02,87.69 R24.1
N$43  (1 unrouted)
N$44
  Top 0.508: IC4.1 77.85,26.42 | 77.85,26.42 77.85,24.77 77.22,24.13 74.99,24.13 R52.2 | R51.2 77.92,26.48 77.85,26.42
N$45  (1 unrouted)
N$46
  Top 0.508: 81.41,71.44 J2.2
  Bottom 1.016: J2.2 85.03,67.95 85.03,58.86 D2.A
  Bottom 2: X4.4 86.36,73.66 86.17,73.47 81.28,73.47 | 81.28,73.47 78.74,73.47 | 78.74,73.47 K2.O | J1.1 78.17,72.9 78.74,73.47 | J2.2 81.53,73.22 81.28,73.47
N$48  (1 unrouted)
  Bottom 0.508: R12.1 44.26,45.66 C6.2 | J3.1 46.29,13.53 46.29,5.78 X6.1
N$50
  Bottom 1.016: 45.09,83.82 45.72,81.28 50.86,75.75 50.8,68.58 50.74,67.37 50.74,57.24 53.34,54.64 53.34,54.55 Q2.1 65.72,54.55 66.55,53.72 66.55,47.05 65.64,46.11 65.47,45.94 arc45 R16.2 | 45.09,83.82 15.24,83.82 12.33,86.73 Q5.1 | Q4.1 45.1,86.37 45.09,83.82
N$51
  Bottom 2: 23.23,86.78 Q5.3 30.3,87.87 R25.1
N$53
  Bottom 0.508: R93.2 69.22,10.86 69.22,7.43 X2.1 70.42,5.08 70.42,3.68 71.12,2.98 82.17,2.98 C91.+
N$54  (1 unrouted)
N$55
  Bottom 0.508: J4.1 53.28,8.89 57.09,5.08 60.83,5.08 60.96,5.21 62.36,5.21 62.94,5.79 P2.1
  Bottom 2: R7-2.2 54.51,26.35 | C57.1 63.92,30.45 arc45 63.63,29.75 C7.- | P2.1 63.4,7.62 arc45 64.11,7.91 65.91,9.72 D11.A 60.36,13.91 arc-45 59.65,14.2 54.36,19.49 R7-2.2 | C7.- 68.74,25.72 arc45 69.44,26.01 R7-1.2 | R7-2.2 56.72,26.35 59.54,23.35 62.89,23.35 63.63,24.34 C7.-
N$56  (1 unrouted)
N$57  (1 unrouted)
N$58  (4 unrouted)
  Top 0.508: IC91.7 87.95,20.83 48.77,20.83 R90.2
V+  (via drill 0.4, 1.3)
  Top 0.508: 55.73,61.85 arc-45 55.88,61.79 | Q2.2 67.06,52.32 68.58,50.8 68.58,46.99 75.92,39.9 77.47,39.9 78.11,39.21 78.11,37.21 82.93,32.45 IC4.3 | 56.01,64.33 55.88,64.45 | v74.87,64.33 62.67,64.33 C1.+
  Top 1.016: 55.82,61.79 55.88,61.79 | 55.88,61.79 55.88,64.45 C1.+ | 55.88,61.79 57.24,60.17 arc-45 57.4,59.15 57.4,54.04 58.1,53.4 60.01,52.2 60.77,52.26 Q2.2 | R13.2 25.4,83.82
  Top 2: v50.48,80.45 40.7,80.45 37.34,83.82 25.4,83.82 20.32,83.82 Q5.2 | B1.+ 56.17,76.33 arc45 55.88,75.63 C1.+
  Bottom 0.508: C1.+ 55.88,81.13 59.05,84.3 R1-2.2 | X3.2 94.23,26.23 90.93,29.53 84.33,29.53 IC4.3 C12.1 | R1.2 75.88,64.33 v74.87,64.33
  Bottom 1.27: C5.1 C1.+
  Bottom 2: 50.51,80.42 50.55,84.9 Q4.2 | 50.51,80.42 v50.48,80.45 | C1.+ 53.63,73.37 arc-45 53.34,74.07 53.34,78.74 51.95,80.13 arc45 51.24,80.42 50.51,80.42
VREF  (1 unrouted)
  Top 0.508: R18.1 16.57,55.63 18.99,58.04 21.97,60.96 23.24,62.23 IC1.6
  Bottom 0.508: R5.1 22.86,70.1 22.23,69.47 | 22.23,69.47 14.41,69.47 12.89,70.99 VR51.2 VR51.1 | 22.23,69.47 22.23,62.99 23.05,62.17 23.11,62.23 IC1.6
VSS  (via drill 0.35, 0.4)
  Top 0.508: v78.3,34.35 78.19,34.39 72.83,34.39 66.65,40.64 v55.88,40.64 | v35.31,61.15 32.26,61.15 IC2.4 31.5,56.39 R14.1 30.92,51.24 30.48,50.8 | 30.48,50.8 27.94,49.15 27.94,48.26 20.32,48.26 IC3.4 | 30.48,50.8 41.53,50.8 44.26,48.07 54.55,48.07 v54.61,48.13
  Bottom 0.508: D7.A 87.19,34.35 v78.3,34.35 | v35.31,61.15 C52.2 | v54.61,48.13 55.88,46.86 v55.88,40.64
  Bottom 1.016: D7.A 92.08,31.69 R3.2

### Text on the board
tNames: Temp. Fühler | AC in / 12V~ | AC in 24V~ | AC in / 12V~ | 30V DC | + Out - | Poti / Spannung | Standby Taster | Standby LED | + Sense - | Poti / Strom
